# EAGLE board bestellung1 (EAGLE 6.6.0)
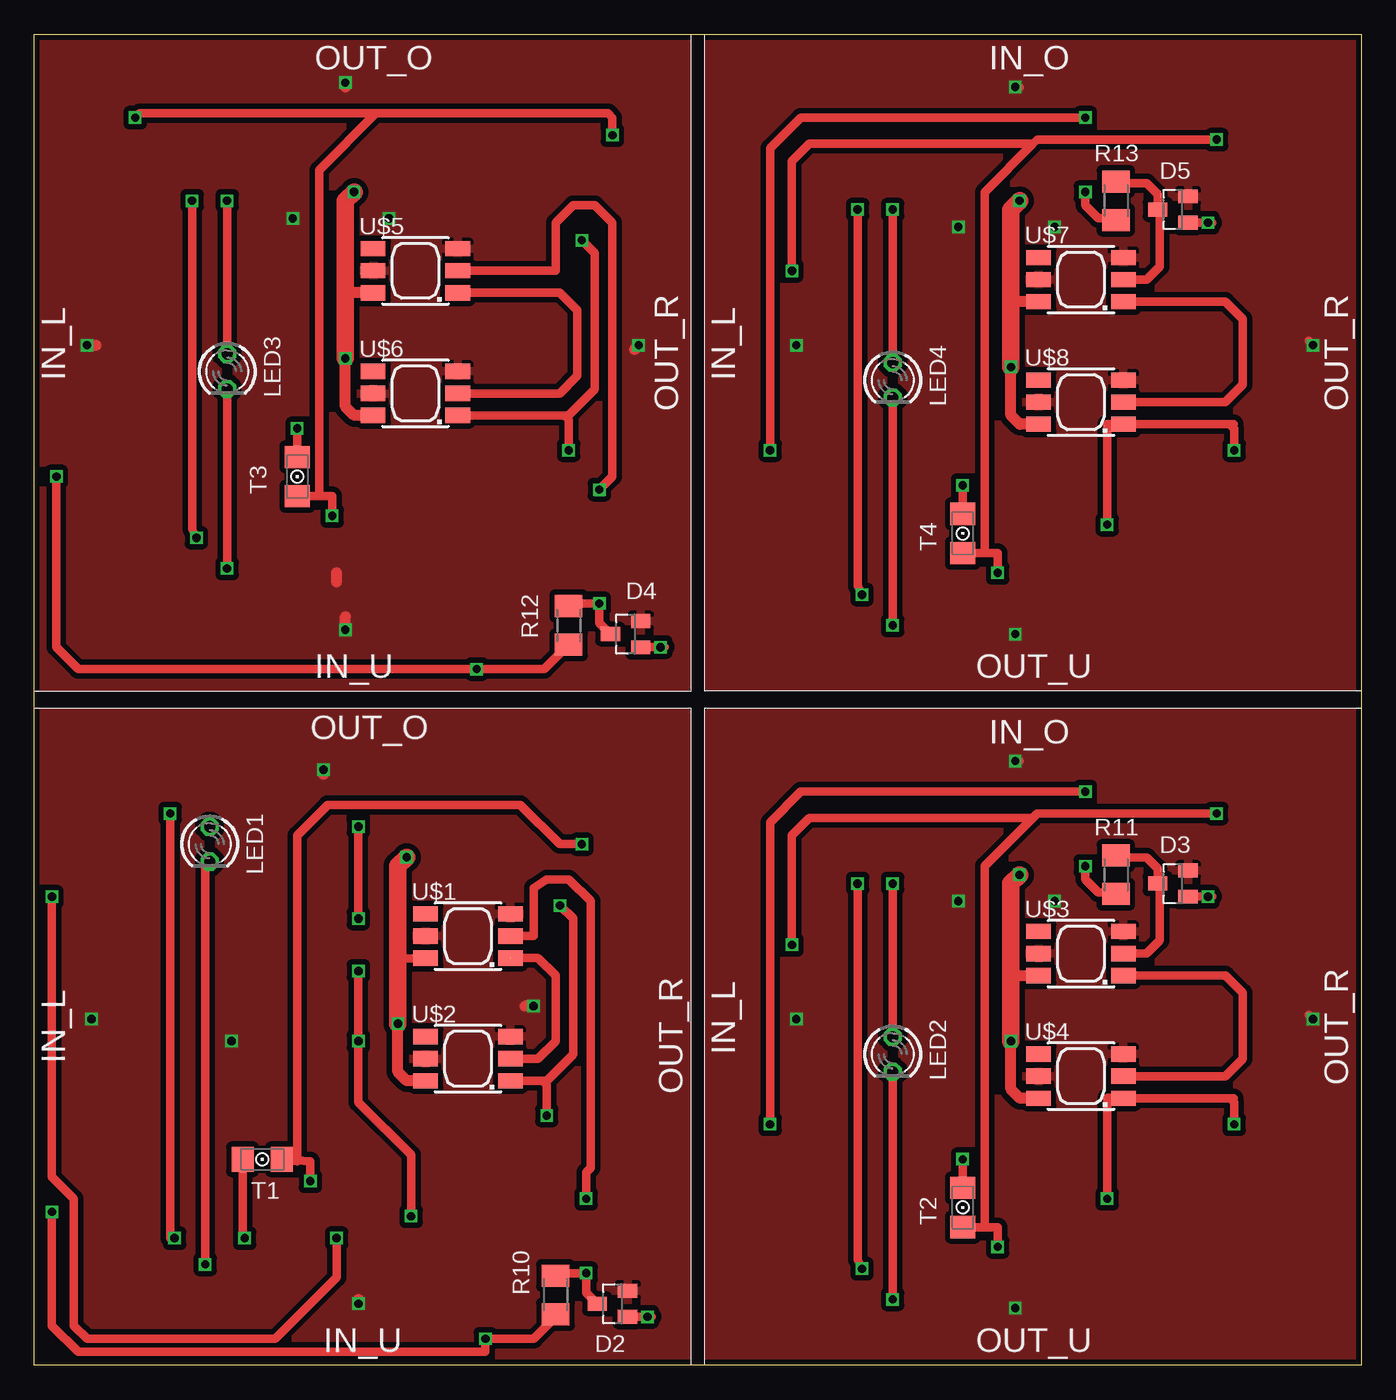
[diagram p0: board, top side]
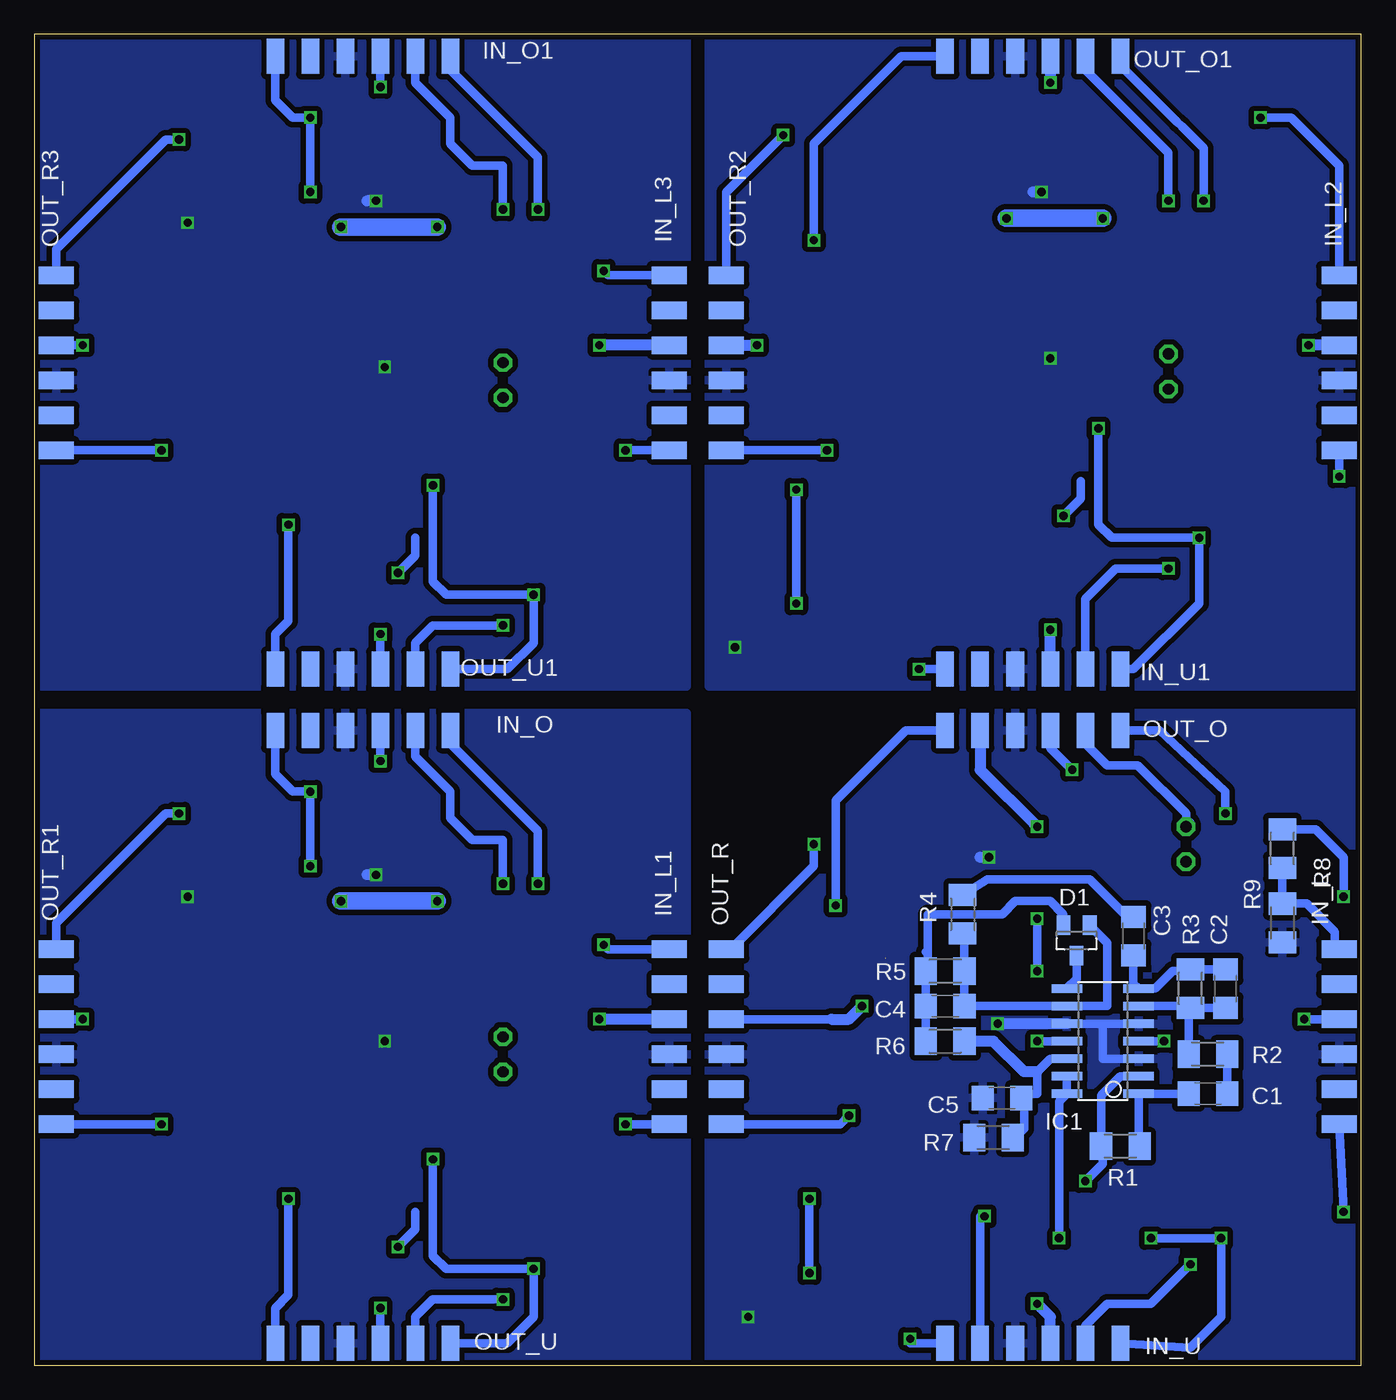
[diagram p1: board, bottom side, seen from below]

Size 96.2 x 96.52 mm. Coordinates in mm from the lower left corner, seen from the top.
Outline: 0,0 0,96.52 96.2,96.52 96.2,0 0,0
Copper layers (1*16): Top 0.035mm / dielectric 1.5mm / Bottom 0.035mm
Design rules "Elecrow_2-layer_eagle_rule": minimum track width 6mil, minimum drill 12mil, track to track 6mil, track to pad 6mil, pad to pad 6mil, via to via 6mil, smd to smd 0mil, copper to edge 10mil, drill to drill 10mil, minimum pad ring 10mil, minimum via ring 6mil, stop-mask expansion 2mil, vias tented up to drill 100mil, thermal gap 10mil

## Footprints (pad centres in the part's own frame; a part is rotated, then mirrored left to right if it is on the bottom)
C1206 = smd 1.6 x 1.8: 1 -1.4,0; 2 1.4,0
SOT23 = smd 1 x 1.4: 1 -0.95,-1.1; 2 0.95,-1.1; 3 0,1.1
SO14 = smd 0.61 x 2.21: 1 -3.81,-2.603; 2 -2.54,-2.603; 3 -1.27,-2.603; 4 0,-2.603; 5 1.27,-2.603; 6 2.54,-2.603; 7 3.81,-2.603; 8 3.81,2.603; 9 2.54,2.603; 10 1.27,2.603; 11 0,2.603; 12 -1.27,2.603; 13 -2.54,2.603; 14 -3.81,2.603
SMD1,27-2,54-6 = smd 1.27 x 2.54: 1 0,0; 2 2.54,0; 3 5.08,0; 4 7.62,0; 5 10.16,0; 6 12.7,0
LED3MM = drill 0.813 octagon: A -1.27,0; K 1.27,0
M1206 = smd 1.6 x 2: 1 -1.4,0; 2 1.4,0
1206 = smd 1.6 x 1.803: A -1.422,0; C 1.422,0
CLN6A = smd 1.778 x 1.1: 1 3.071,-1.6; 2 3.071,0; 3 3.071,1.6; 4 -3.071,1.6; 5 -3.071,0; 6 -3.071,-1.6

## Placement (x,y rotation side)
C1  [C1206]  11.11,19.68 0 bottom
C2  [C1206]  9.84,27.3 90 bottom
C3  [C1206]  16.51,31.11 90 bottom
C4  [C1206]  30.16,26.04 180 bottom
C5  [C1206]  26.04,19.37 0 bottom
D1  BAS40-04  [SOT23]  20.64,30.8 180 bottom
D2  BAS40-04  [SOT23]  41.91,4.45 90 top
D3  BAS40-04  [SOT23]  82.55,34.92 90 top
D4  BAS40-04  [SOT23]  42.86,53.02 90 top
D5  BAS40-04  [SOT23]  82.55,83.82 90 top
IC1  LM837U  [SO14]  18.73,23.5 90 bottom
IN_L  SMD2-6  [SMD1,27-2,54-6]  1.59,30.16 270 bottom
IN_L1  SMD2-6  [SMD1,27-2,54-6]  50.16,30.16 270 bottom
IN_L2  SMD2-6  [SMD1,27-2,54-6]  1.59,79.06 270 bottom
IN_L3  SMD2-6  [SMD1,27-2,54-6]  50.16,79.06 270 bottom
IN_O  SMD2-6  [SMD1,27-2,54-6]  66.04,46.04 180 bottom
IN_O1  SMD2-6  [SMD1,27-2,54-6]  66.04,94.93 180 bottom
IN_U  SMD2-6  [SMD1,27-2,54-6]  17.46,1.59 180 bottom
IN_U1  SMD2-6  [SMD1,27-2,54-6]  17.46,50.48 180 bottom
LED1  [LED3MM]  12.7,37.78 270 top
LED2  [LED3MM]  62.23,22.54 270 top
LED3  [LED3MM]  13.97,72.07 270 top
LED4  [LED3MM]  62.23,71.44 270 top
OUT_O  SMD2-6  [SMD1,27-2,54-6]  17.46,46.04 180 bottom
OUT_O1  SMD2-6  [SMD1,27-2,54-6]  17.46,94.93 180 bottom
OUT_R  SMD2-6  [SMD1,27-2,54-6]  46.04,30.16 270 bottom
OUT_R1  SMD2-6  [SMD1,27-2,54-6]  94.61,30.16 270 bottom
OUT_R2  SMD2-6  [SMD1,27-2,54-6]  46.04,79.06 270 bottom
OUT_R3  SMD2-6  [SMD1,27-2,54-6]  94.61,79.06 270 bottom
OUT_U  SMD2-6  [SMD1,27-2,54-6]  66.04,1.59 180 bottom
OUT_U1  SMD2-6  [SMD1,27-2,54-6]  66.04,50.48 180 bottom
R1  [M1206]  17.46,15.88 0 bottom
R2  [M1206]  11.11,22.54 0 bottom
R3  [M1206]  12.38,27.3 270 bottom
R4  [M1206]  28.89,32.7 90 bottom
R5  [M1206]  30.16,28.57 0 bottom
R6  [M1206]  30.16,23.5 180 bottom
R7  [M1206]  26.67,16.51 180 bottom
R8  [M1206]  5.71,37.47 270 bottom
R9  [M1206]  5.71,32.07 90 bottom
R10  [M1206]  37.78,5.08 90 top
R11  [M1206]  78.42,35.56 90 top
R12  [M1206]  38.73,53.66 90 top
R13  [M1206]  78.42,84.45 90 top
T1  PHOTO-TRANS-1206  [1206]  16.51,14.92 180 top
T2  PHOTO-TRANS-1206  [1206]  67.31,11.43 90 top
T3  PHOTO-TRANS-1206  [1206]  19.05,64.45 90 top
T4  PHOTO-TRANS-1206  [1206]  67.31,60.33 90 top
U$1  LED_SMD5050  [CLN6A]  31.43,31.11 0 top
U$2  LED_SMD5050  [CLN6A]  31.43,22.23 0 top
U$3  LED_SMD5050  [CLN6A]  75.88,29.84 0 top
U$4  LED_SMD5050  [CLN6A]  75.88,20.95 0 top
U$5  LED_SMD5050  [CLN6A]  27.62,79.38 0 top
U$6  LED_SMD5050  [CLN6A]  27.62,70.48 0 top
U$7  LED_SMD5050  [CLN6A]  75.88,78.74 0 top
U$8  LED_SMD5050  [CLN6A]  75.88,69.85 0 top

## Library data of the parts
C1-C5 R1-R13 = resistor
D1-D5 = diode
IC1 = #mylib; OC_FARNELL: unknown; OC_NEWARK: unknown
IN_L IN_L1-IN_L3 IN_O IN_O1 IN_U IN_U1 OUT_O OUT_O1 OUT_R OUT_R1-OUT_R3 OUT_U OUT_U1 T1-T4 U$1-U$8 = #mylib
LED1-LED4 = led

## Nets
+5V: D2.2 IC1.4 IN_L.3 IN_U.3 OUT_O.3 OUT_R.3 U$1.3 U$1.5 U$2.3 U$2.5
+5V1: D3.2 IN_L1.3 IN_O.3 OUT_R1.3 OUT_U.3 U$3.3 U$3.5 U$4.3 U$4.5
+5V2: D4.2 IN_L2.3 IN_U1.3 OUT_O1.3 OUT_R2.3 U$5.3 U$5.5 U$6.3 U$6.5
+5V3: D5.2 IN_L3.3 IN_O1.3 OUT_R3.3 OUT_U1.3 U$7.3 U$7.5 U$8.3 U$8.5
-5V: IC1.11 IN_U.5 OUT_O.5
GND: C5.1 D2.1 IC1.3 IC1.5 IC1.10 IN_L.4 IN_U.4 OUT_O.4 OUT_R.4 R7.2 R9.1 U$1.6 U$2.6
GND1: D3.1 IN_L1.4 IN_O.4 OUT_R1.4 OUT_U.4 U$3.6 U$4.6
GND2: D4.1 IN_L2.4 IN_U1.4 OUT_O1.4 OUT_R2.4 U$5.6 U$6.6
GND3: D5.1 IN_L3.4 IN_O1.4 OUT_R3.4 OUT_U1.4 U$7.6 U$8.6
N$1: IC1.2 OUT_R.1 R1.1 T1.A
N$2: C1.1 IC1.1 R1.2
N$3: C1.2 R2.2
N$4: IN_U.1 OUT_O.1 T1.C
N$5: D1.3 IC1.8
N$6: U$1.1 U$2.2
N$7: D2.3 R10.2 U$1.2
N$8: IC1.13 IC1.14 R8.1
N$9: C2.1 IC1.6 R2.1 R3.2
N$10: C2.2 C3.1 IC1.7 R3.1
N$11: C4.2 D1.2 R5.1 R6.2
N$12: U$3.1 U$4.2
N$13: LED1.A OUT_O.2
N$14: C3.2 R4.2
N$15: C4.1 D1.1 IC1.9 R4.1 R5.2
N$16: IN_O.1 OUT_U.1 T2.C
N$17: IN_L.6 IN_U.6 R10.1
N$18: IN_L.1 R8.2 R9.2
N$19: C5.2 IC1.12 R6.1 R7.1
N$20: IN_O.2 LED2.A
N$21: OUT_O.6 OUT_R.6 U$2.1
N$22: LED2.K OUT_U.2
N$23: IN_L1.6 IN_O.6 R11.1
N$24: IN_L1.1 OUT_R1.1 T2.A
N$25: IN_U.2 LED1.K
N$26: D3.3 R11.2 U$3.2
N$27: OUT_R1.6 OUT_U.6 U$4.1
N$28: U$5.1 U$6.2
N$29: IN_U1.1 OUT_O1.1 T3.C
N$30: LED3.A OUT_O1.2
N$31: IN_U1.2 LED3.K
N$32: IN_L2.6 IN_U1.6 R12.1
N$33: IN_L2.1 OUT_R2.1 T3.A
N$34: D4.3 R12.2 U$5.2
N$35: OUT_O1.6 OUT_R2.6 U$6.1
N$36: U$7.1 U$8.2
N$37: IN_O1.1 OUT_U1.1 T4.C
N$38: IN_O1.2 LED4.A
N$39: LED4.K OUT_U1.2
N$40: IN_L3.6 IN_O1.6 R13.1
N$41: IN_L3.1 OUT_R3.1 T4.A
N$42: D5.3 R13.2 U$7.2
N$43: OUT_R3.6 OUT_U1.6 U$8.1

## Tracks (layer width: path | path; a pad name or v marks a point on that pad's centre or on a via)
+5V  (via drill 0.6)
  Top 0.813: v20.95,43.18 20.95,42.86 | v36.2,26.04 35.56,26.04 | v23.5,4.45 23.5,4.76
  Bottom 0.61: IN_L.3 v4.13,25.08 | OUT_R.3 38.42,25.08 | v14.29,23.5 IC1.4 | OUT_O.3 22.54,44.77 v20.95,43.18
  Bottom 0.813: 38.42,25.08 37.15,25.08 v36.2,26.04 | IN_U.3 22.54,3.49 v23.5,4.45
  pour Top (isolate 0.406): 0.32,47.31 47.31,47.31 47.31,0.32 0.32,0.32
+5V1  (via drill 0.6)
  Top 0.61: v71.12,43.81 71.44,43.81 | v92.71,25.08 92.39,25.4
  Bottom 0.61: IN_O.3 v71.12,43.81 | OUT_R1.3 v92.71,25.08 | v71.12,4.13 OUT_U.3
  Bottom 0.813: IN_L1.3 v55.24,25.08
  Bottom 1.27: v66.99,33.66 v73.98,33.66
  pour Top (isolate 0.406): 48.9,47.31 95.89,47.31 95.89,0.32 48.9,0.32
+5V2  (via drill 0.6)
  Top 0.813: 21.91,56.83 21.91,57.47 | v43.81,73.98 43.5,73.66 | v22.54,53.34 22.54,54.29 | v3.81,73.98 4.45,73.98 | v22.54,93.03 22.54,92.71
  Bottom 0.813: OUT_R2.3 v43.81,73.98 | IN_U1.3 v22.54,53.34 | IN_L2.3 v3.81,73.98 | OUT_O1.3 v22.54,93.03
  Bottom 1.27: v18.73,83.19 v25.72,83.19
  pour Top (isolate 0.406): 0.32,96.2 47.31,96.2 47.31,49.21 0.32,49.21
+5V3  (via drill 0.6)
  Top 0.61: v71.12,92.71 71.44,92.71 | v92.71,73.98 92.39,74.3
  Bottom 0.61: IN_O1.3 v71.12,92.71 | OUT_R3.3 v92.71,73.98 | v71.12,53.02 OUT_U1.3
  Bottom 0.813: IN_L3.3 v55.24,73.98
  Bottom 1.27: v66.99,82.55 v73.98,82.55
  pour Top (isolate 0.406): 48.9,96.2 95.89,96.2 95.89,49.21 48.9,49.21
-5V  (via drill 0.6)
  Top 0.61: v27.3,10.79 27.3,15.24 23.5,19.05 v23.5,23.5 v23.5,28.57 | v23.5,39.05 v23.5,32.38
  Bottom 0.61: IC1.11 v23.5,23.5 | v23.5,32.38 v23.5,28.57 | IN_U.5 27.62,10.79 v27.3,10.79
  Bottom 0.813: 23.81,39.37 v23.5,39.05 27.62,43.18 OUT_O.5
GND  (via drill 0.6)
  Top 0.61: D2.1 44.77,3.5 v44.45,3.49 | U$1.6 26.36,29.52
  Top 0.813: U$2.6 27,20.62 26.35,21.27 v26.35,24.77 | 26.36,29.52 26.35,29.53
  Top 1.27: v26.35,24.77 26.35,29.53 26.35,36.2 v26.99,36.83
  Bottom 0.61: IC1.10 18.73,24.77 | 18.73,24.77 IC1.5 | IC1.3 18.73,22.23 18.73,24.77
  Bottom 0.813: v26.99,36.83 27.62,36.83 | IC1.10 v26.35,24.77
  pour Bottom (isolate 0.406): 0.32,47.31 47.31,47.31 47.31,0.32 0.32,0.32
GND1  (via drill 0.6)
  Top 0.61: D3.1 85.41,33.98 v85.09,33.97
  Top 0.813: U$4.6 71.45,19.36 70.8,20 v70.8,23.5 | U$3.6 70.81,28.25 70.8,28.26
  Top 1.27: v70.8,23.5 70.8,28.26 70.8,34.92 v71.44,35.56
  Bottom 0.813: v71.44,35.56 72.07,35.56
  pour Bottom (isolate 0.406): 48.9,47.31 95.89,47.31 95.89,0.32 48.9,0.32
GND2  (via drill 0.6)
  Top 0.61: D4.1 45.72,52.07 v45.4,52.07
  Top 0.813: U$6.6 23.19,68.89 22.54,69.53 v22.54,73.03 | U$5.6 22.55,77.78 22.54,77.79
  Top 1.27: v22.54,73.03 22.54,77.79 22.54,84.45 v23.18,85.09
  Bottom 0.813: v23.18,85.09 23.81,85.09
  pour Bottom (isolate 0.406): 0.32,96.2 47.31,96.2 47.31,49.21 0.32,49.21
GND3  (via drill 0.6)
  Top 0.61: D5.1 85.41,82.87 v85.09,82.87
  Top 0.813: U$8.6 71.45,68.25 70.8,68.9 v70.8,72.39 | U$7.6 70.81,77.14 70.8,77.15
  Top 1.27: v70.8,72.39 70.8,77.15 70.8,83.82 v71.44,84.45
  Bottom 0.813: v71.44,84.45 72.07,84.45
  pour Bottom (isolate 0.406): 48.9,96.2 95.89,96.2 95.89,49.21 48.9,49.21
N$1  (via drill 0.6)
  Top 0.61: v20,13.34 20,14.77 T1.A 19.05,14.77 19.05,38.42 21.27,40.64 35.24,40.64 38.1,37.78 v39.69,37.78
  Bottom 0.61: IC1.2 17.46,20.95 18.86,19.55 R1.1 18.73,15.88 18.73,14.61 v20,13.34 | OUT_R.1 45.72,30.16 39.69,36.2 v39.69,37.78
N$2
  Bottom 0.61: C1.1 IC1.1 16.13,15.94 R1.2
N$3
  Bottom 0.61: C1.2 R2.2
N$4  (via drill 0.6)
  Top 0.61: v9.84,40.01 9.84,9.21 v10.16,9.21 | T1.C 15.09,9.36 v15.24,9.21
  Bottom 0.61: v15.24,9.21 v10.16,9.21 10.16,3.49 12.38,1.27 IN_U.1 | v9.84,40.01 9.84,41.59 14.61,46.04 OUT_O.1
N$5
  Bottom 0.61: 21.27,27.37 IC1.8 20.64,28 D1.3
N$6  (1 unrouted)
  Top 0.61: U$2.2 36.51,22.23 37.78,23.5 37.78,28.26 36.51,29.53 34.52,29.53
N$7  (via drill 0.6)
  Top 0.61: 40.96,4.3 D2.3 40.01,5.25 v40.01,6.67 37.97,6.67 R10.2 | v40.01,12.06 40.01,13.97 40.32,14.29 40.32,33.66 38.73,35.24 37.15,35.24 36.2,34.61 36.2,31.11 U$1.2
  Bottom 0.61: v40.01,6.67 v40.01,12.06
N$8  (via drill 0.6)
  Top 0.61: v1.27,33.97 1.27,13.65 2.86,12.06 2.86,2.86 3.81,1.91 17.46,1.91 21.91,6.35 v21.91,9.21
  Bottom 0.61: IC1.13 IC1.14 21.91,19.11 v21.91,9.21 | R8.1 3.31,38.87 1.27,36.83 v1.27,33.97
N$9
  Bottom 0.61: IC1.6 12.51,26.04 R3.2 | R3.2 C2.1 | R2.1 12.51,25.77 R3.2
N$10
  Bottom 0.61: C2.2 R3.1 12.51,28.57 13.65,28.57 14.92,27.3 IC1.7 16.51,27.69 C3.1
N$11
  Bottom 0.61: 31.69,26.16 C4.2 | C4.2 R5.1 31.43,28.7 31.43,29.84 | 31.43,29.84 31.43,32.7 26.04,32.7 25.08,33.66 22.54,33.66 21.59,32.7 D1.2 | 31.56,29.98 31.43,29.84 | C4.2 R6.2
N$12
  Top 0.61: U$4.2 86.36,20.95 87.63,22.23 87.63,26.99 86.36,28.26 78.97,28.26 U$3.1
N$13
  Bottom 0.61: 12.38,39.37 LED1.A 12.7,40.01 16.19,43.5 18.41,43.5 20,45.09 OUT_O.2
N$14
  Bottom 0.61: R4.2 27.12,35.24 19.68,35.24 16.96,32.52 C3.2
N$15
  Bottom 0.61: R4.1 28.76,30.86 R5.2 C4.1 IC1.9 18.41,26.04 18.41,30.62 D1.1
N$16  (via drill 0.6)
  Top 0.61: v59.69,34.92 59.69,7.62 v60.01,6.99 | v67.31,14.92 T2.C
  Bottom 0.61: v59.69,34.92 59.69,38.73 66.04,45.09 IN_O.1 | v67.31,14.92 67.31,7.94 66.36,6.99 v60.01,6.99 60.01,3.49 61.91,1.59 OUT_U.1
N$17  (via drill 0.6)
  Top 0.61: R10.1 37.78,3.49 36.2,1.91 v32.7,1.91 32.7,0.95 3.17,0.95 1.27,2.86 v1.27,11.11
  Bottom 0.61: v1.27,11.11 IN_L.6 | IN_U.6 32.7,1.59 v32.7,1.91
N$18
  Bottom 0.61: R8.2 R9.2 3.94,33.47 1.91,31.43 1.91,30.48 IN_L.1
N$19
  Bottom 0.61: IC1.12 22.54,22.23 23.5,21.27 23.5,19.68 24.32,19.68 C5.2 | 24.45,19.55 C5.2 | 25.27,16.7 R7.1 25.08,16.51 24.45,17.14 24.45,19.18 C5.2
  Bottom 0.813: 23.5,21.27 24.45,21.27 26.67,23.5 R6.1
N$20  (via drill 0.6)
  Top 0.61: v62.23,34.92 LED2.A
  Bottom 0.61: v62.23,34.92 62.23,38.1 64.45,38.1 66.04,39.69 66.04,41.59 68.58,44.13 IN_O.2
N$21  (via drill 0.6)
  Top 0.61: U$2.1 36.83,20.62 | 36.83,20.62 37.13,20.62 39.05,22.54 39.05,32.38 v38.1,33.34 | v37.15,18.1 37.15,20.31 36.83,20.62
  Bottom 0.61: v38.1,33.34 38.1,40.96 33.02,46.04 OUT_O.6 | OUT_R.6 37.78,17.46 v37.15,18.1
N$22  (via drill 0.6)
  Top 0.61: v62.23,4.76 LED2.K
  Bottom 0.61: OUT_U.2 68.58,3.49 67.31,4.76 v62.23,4.76
N$23  (via drill 0.6)
  Top 0.61: v76.2,36.2 76.2,35.24 77.15,34.29 78.29,34.29 R11.1 | v53.34,17.46 53.34,39.37 55.56,41.59 v76.2,41.59
  Bottom 0.61: v76.2,36.2 v76.2,41.59 77.47,41.59 78.74,42.86 IN_O.6 | IN_L1.6 v53.34,17.46
N$24  (via drill 0.6)
  Top 0.61: v69.85,8.57 69.85,10.01 68.9,10.01 | 72.39,39.69 72.71,40.01 v85.72,40.01 | 72.39,39.69 68.9,36.2 68.9,10.01 | 68.9,10.01 T2.A | v54.93,30.48 54.93,38.42 56.2,39.69 72.39,39.69
  Bottom 0.61: 68.58,11.11 68.58,9.84 v69.85,8.57 | v85.72,40.01 86.68,40.01 94.61,32.07 OUT_R1.1 | IN_L1.1 54.61,30.16 v54.93,30.48
N$25  (via drill 0.6)
  Top 0.61: v12.38,7.3 12.38,36.2 LED1.K
  Bottom 0.61: IN_U.2 20,2.86 18.41,4.45 15.24,4.45 v12.38,7.3
N$26
  Top 0.61: U$3.2 80.64,29.84 81.6,30.8 81.6,34.78 D3.3 81.45,36.02 80.64,36.83 78.55,36.83 R11.2
N$27  (via drill 0.6)
  Top 0.61: 86.68,19.36 U$4.1 78.95,19.37 77.79,19.37 v77.79,12.06 | 86.68,19.36 86.98,19.36 | v87,17.46 87,19.04 86.68,19.36
  Bottom 0.61: OUT_R1.6 v87,17.46 | v77.79,12.06 77.79,5.08 78.74,4.13 OUT_U.6
N$28
  Top 0.61: U$6.2 38.1,70.48 39.37,71.75 39.37,76.52 38.1,77.79 30.71,77.79 U$5.1
N$29  (via drill 0.6)
  Top 0.61: v11.43,84.45 11.43,60.64 v11.75,60.01 | v19.05,67.94 T3.C
  Bottom 0.61: v11.43,84.45 11.43,88.27 13.02,89.85 13.34,90.17 17.46,94.3 OUT_O1.1 | v19.05,67.94 19.05,60.96 18.1,60.01 v11.75,60.01 11.75,55.24 16.51,50.48 IN_U1.1
N$30  (via drill 0.6)
  Top 0.61: v13.97,84.45 LED3.A
  Bottom 0.61: v13.97,84.45 13.97,87.95 20,93.98 OUT_O1.2
N$31  (via drill 0.6)
  Top 0.61: v13.97,57.78 LED3.K
  Bottom 0.61: v13.97,57.78 17.78,57.78 20,55.56 IN_U1.2
N$32  (via drill 0.6)
  Top 0.61: R12.1 36.96,50.48 v32.07,50.48 3.17,50.48 1.59,52.07 v1.59,64.45
  Bottom 0.61: IN_U1.6 v32.07,50.48 | IN_L2.6 v1.59,64.45
N$33  (via drill 0.6)
  Top 0.61: v21.59,61.59 21.59,63.03 T3.A 20.64,63.03 20.64,86.68 24.77,90.81 | v41.91,89.22 41.91,90.49 41.59,90.81 24.77,90.81 | v7.3,90.49 7.62,90.81 24.77,90.81
  Bottom 0.61: 20.32,64.14 20.32,62.87 v21.59,61.59 | OUT_R2.1 46.04,85.09 v41.91,89.22 | v7.3,90.49 5.08,90.49 1.59,87 IN_L2.1
N$34  (via drill 0.6)
  Top 0.61: 41.91,52.88 D4.3 40.96,53.83 v40.96,55.24 38.92,55.24 R12.2 | U$5.2 37.78,79.38 37.78,82.87 39.05,84.14 40.64,84.14 41.91,82.87 41.91,64.45 v40.96,63.5
  Bottom 0.61: v40.96,55.24 v40.96,63.5
N$35  (via drill 0.6)
  Top 0.61: U$6.1 38.42,68.89 | 38.42,68.89 38.72,68.89 40.64,70.8 40.64,80.64 v39.69,81.6 | v38.73,66.36 38.73,68.57 38.42,68.89
  Bottom 0.61: v39.69,81.6 39.69,88.58 33.34,94.93 OUT_O1.6 | OUT_R2.6 v38.73,66.36
N$36
  Top 0.61: U$8.2 86.36,69.85 87.63,71.12 87.63,75.88 86.36,77.15 78.97,77.15 U$7.1
N$37  (via drill 0.6)
  Top 0.61: v59.69,83.82 59.69,56.52 v60.01,55.88 | v67.31,63.82 T4.C
  Bottom 0.61: v59.69,83.82 59.69,87.63 66.04,93.98 IN_O1.1 | v67.31,63.82 67.31,56.83 66.36,55.88 v60.01,55.88 60.01,52.39 61.91,50.48 OUT_U1.1
N$38  (via drill 0.6)
  Top 0.61: v62.23,83.82 LED4.A
  Bottom 0.61: v62.23,83.82 62.23,87 64.45,87 66.04,88.58 66.04,90.49 68.58,93.03 IN_O1.2
N$39  (via drill 0.6)
  Top 0.61: v62.23,53.66 LED4.K
  Bottom 0.61: OUT_U1.2 68.58,52.39 67.31,53.66 v62.23,53.66
N$40  (via drill 0.6)
  Top 0.61: v76.2,85.09 76.2,84.14 77.15,83.19 78.29,83.19 R13.1 | v53.34,66.36 53.34,88.27 55.56,90.49 v76.2,90.49
  Bottom 0.61: v76.2,85.09 v76.2,90.49 77.47,90.49 78.74,91.76 IN_O1.6 | IN_L3.6 v53.34,66.36
N$41  (via drill 0.6)
  Top 0.61: v69.85,57.47 69.85,58.9 68.9,58.9 | 72.39,88.58 72.71,88.9 v85.72,88.9 | 72.39,88.58 68.9,85.09 68.9,58.9 | 68.9,58.9 T4.A | v54.93,79.38 54.93,87.31 56.2,88.58 72.39,88.58
  Bottom 0.61: 68.58,60.01 68.58,58.74 v69.85,57.47 | v85.72,88.9 86.68,88.9 94.61,80.96 OUT_R3.1 | IN_L3.1 54.61,79.06 v54.93,79.38
N$42
  Top 0.61: U$7.2 80.64,78.74 81.6,79.69 81.6,83.67 D5.3 81.45,84.92 80.64,85.72 78.55,85.72 R13.2
N$43  (via drill 0.6)
  Top 0.61: 86.68,68.25 U$8.1 78.95,68.26 77.79,68.26 v77.79,60.96 | 86.68,68.25 86.98,68.25 | v87,66.36 87,67.93 86.68,68.25
  Bottom 0.61: OUT_R3.6 v87,66.36 | v77.79,60.96 77.79,53.98 78.74,53.02 OUT_U1.6

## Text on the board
tNames: OUT_O | IN_O | IN_L | IN_L | OUT_R | OUT_R | IN_U | OUT_U | OUT_O | IN_O | IN_L | IN_L | OUT_R | OUT_R | IN_U | OUT_U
